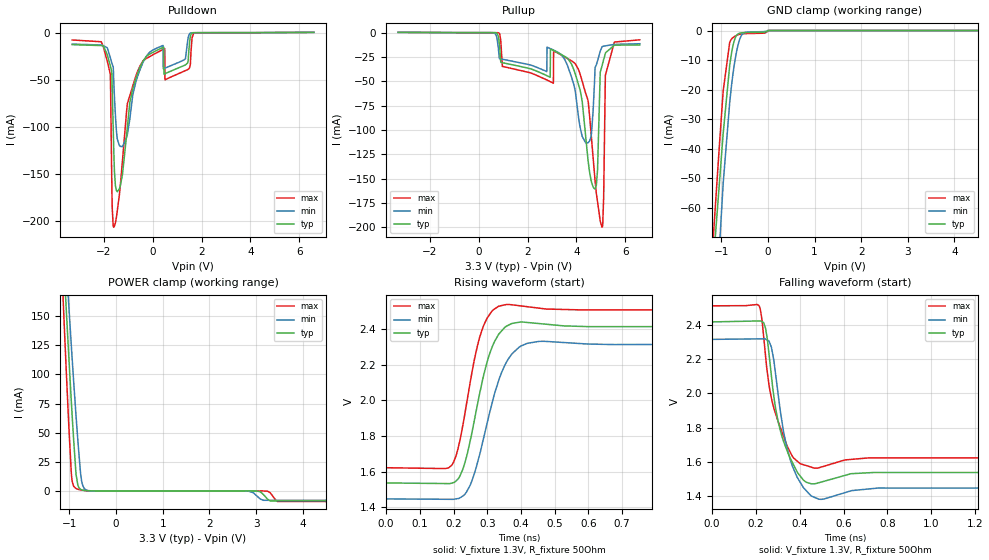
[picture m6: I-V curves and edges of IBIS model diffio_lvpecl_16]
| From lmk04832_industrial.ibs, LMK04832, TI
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|   diffio_lvpecl_16 Model
[Model]   diffio_lvpecl_16
Model_type   I/O
Polarity   Non-Inverting
Enable   Active-High
Vinl = 0.4
Vinh = 1.2
Vmeas = 2
Vref = 1.3
Cref = 1pF
Rref = 50
|   typ   min   max
C_comp   1.613pF   1.569pF   1.681pF
|  Where Nom  PVT is Nominal Process,   3.3V,  25C
|   Fast PVT is Strong Process,   3.45V, -40C
|   Slow PVT is Weak Process,   3.15V, 85C
[Model spec]
|subparameter
Vinl   0.400   0.370   0.430
Vinh   1.200   1.170   1.230
[Voltage Range]   3.3   3.15   3.45
|Junction Temperature
[Temperature Range]   25   85   -40
[Pullup Reference]   3.3   3.15   3.45
[Pulldown Reference]   0   0   0
[Power Clamp Reference]   3.3   3.15   3.45
[GND Clamp Reference]   0   0   0
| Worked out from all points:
|   GND clamp passes 1 mA (typ) near -0.62 V on its own axis
|   POWER clamp passes 1 mA (typ) near -0.74 V on its own axis
|   falling waveform, V_fixture 1.3V, R_fixture 50Ohm: 20-80 % time 69.4ps typ, 68.4ps min, 76.5ps max; typ from 2.42 V to 1.54 V
|   rising waveform, V_fixture 1.3V, R_fixture 50Ohm: 20-80 % time 61.1ps typ, 72.5ps min, 52.8ps max; typ from 1.54 V to 2.42 V
[Pulldown]
|   Voltage   I(typ)   I(min)   I(max)
-3.3V     -12.72mA   -12.09mA   -7.755mA
-2.11V    -13.67mA   -13.08mA   -9.631mA
-1.74V    -35.09mA   -26.45mA   -43.95mA
-1.66V    -61.58mA   -33.59mA   -186.5mA
-1.6V     -122.6mA   -49.83mA   -206mA
-1.49V    -167.2mA   -104mA     -195.6mA
-1.24V    -149.8mA   -120.6mA   -135mA
-1.04V    -99.67mA   -107.4mA   -75.03mA
-390mV    -29.74mA   -30.98mA   -29.68mA
500mV     -43.46mA   -37.6mA    -50mA
1.68V     -68.85uA   -43.61uA   -276.3uA
6.6V      322.5uA    295.4uA    354.8uA
[GND Clamp]
|   Voltage   I(typ)   I(min)   I(max)
-3.3V     -880.2mA   -824.9mA   -955.5mA
-1.18V    -80.5mA    -122.1mA   -71.85mA
-1.04V    -51.39mA   -73.25mA   -38.58mA
-960mV    -34.84mA   -51.71mA   -20.4mA
-820mV    -11.74mA   -24.32mA   -3.983mA
-730mV    -3.862mA   -12.43mA   -2.166mA
-670mV    -1.608mA   -6.896mA   -1.634mA
-620mV    -991.5uA   -3.63mA    -1.335mA
-570mV    -794.2uA   -1.677mA   -1.162mA
-500mV    -706.1uA   -676.8uA   -1.062mA
0V        0A         0A         0A
6.6V      0A         0A         0A
[Pullup]
|   Voltage   I(typ)   I(min)   I(max)
-3.3V     316.7uA    286.1uA    320.8uA
800mV     -3.304mA   -14.79mA   -99.19uA
970mV     -30.83mA   -27.3mA    -34.7mA
2.8V      -44.23mA   -14.9mA    -48.66mA
3.9V      -38.21mA   -53.59mA   -30.63mA
4.48V     -130.8mA   -113mA     -69.67mA
4.76V     -160.4mA   -40.82mA   -149.4mA
4.87V     -140.9mA   -29.01mA   -173.6mA
5.06V     -33.48mA   -14.51mA   -199.7mA
5.12V     -27.59mA   -13.88mA   -169.4mA
5.19V     -21.44mA   -13.56mA   -43.94mA
6.6V      -12.65mA   -11.4mA    -7.381mA
[POWER Clamp]
|   Voltage   I(typ)   I(min)   I(max)
-3.3V     1.944A     1.741A     2.257A
-1.23V    279.5mA    301.8mA    251.5mA
-1.11V    186.9mA    221.6mA    140.1mA
-1.07V    156.6mA    195.3mA    104.1mA
-1.01V    112.1mA    156.2mA    52.47mA
-960mV    76.51mA    124.5mA    14.98mA
-920mV    49.82mA    99.77mA    4.868mA
-860mV    14.5mA     64.71mA    2.062mA
-820mV    4.859mA    43.26mA    1.488mA
-740mV    963.9uA    8.663mA    758.6uA
-610mV    149uA      399.9uA    139uA
6.6V      -8.594mA   -8.021mA   -9.078mA
[Ramp]
R_load = 50
|   typ   min   max
dV/dt_r   0.528402/6.1146e-11   0.520614/7.251e-11   0.533323/5.27774e-11
dV/dt_f   0.528346/6.88763e-11   0.521807/6.78678e-11   0.533237/7.61536e-11
[Falling Waveform]
V_fixture = 1.3V
V_fixture_min = 1.15V
V_fixture_max = 1.45V
R_fixture = 50Ohm
C_fixture = 0F
|   Time   V(typ)   V(min)   V(max)
0s        2.418V     2.316V     2.512V
214ps     2.423V     2.319V     2.514V
244.4ps   2.379V     2.317V     2.217V
260.1ps   2.231V     2.306V     2.049V
289.8ps   1.916V     2.116V     1.883V
326ps     1.722V     1.781V     1.752V
388.5ps   1.542V     1.511V     1.605V
466ps     1.473V     1.394V     1.564V
739.7ps   1.539V     1.446V     1.624V
10ns      1.537V     1.446V     1.623V
[Rising Waveform]
V_fixture = 1.3V
V_fixture_min = 1.15V
V_fixture_max = 1.45V
R_fixture = 50Ohm
C_fixture = 0F
|   Time   V(typ)   V(min)   V(max)
0s        1.536V     1.447V     1.622V
185.6ps   1.533V     1.445V     1.621V
212.6ps   1.556V     1.449V     1.724V
249ps     1.769V     1.522V     2.097V
283.9ps   2.095V     1.745V     2.393V
317.9ps   2.315V     2.011V     2.509V
356.9ps   2.417V     2.215V     2.539V
400.3ps   2.44V      2.306V     2.531V
469.1ps   2.429V     2.332V     2.514V
10ns      2.417V     2.314V     2.511V
